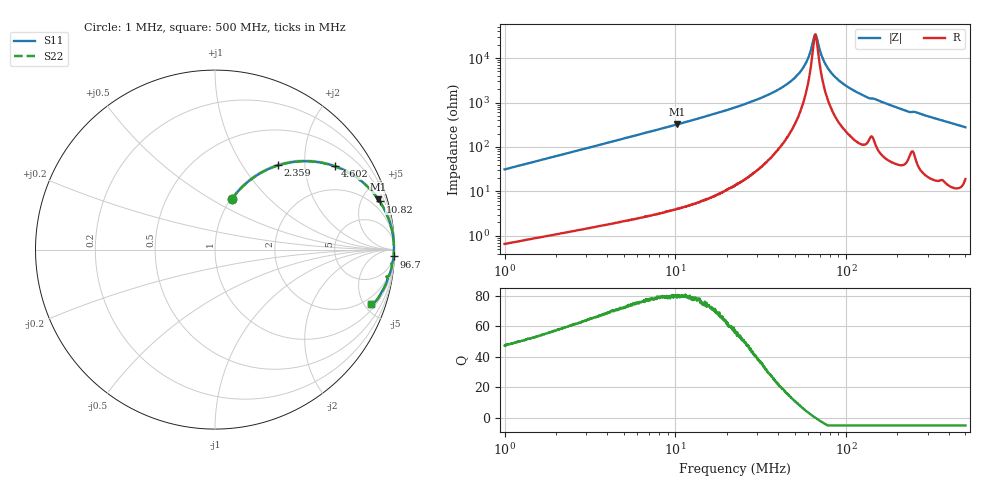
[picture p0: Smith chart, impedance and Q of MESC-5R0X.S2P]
!s-Parameter Generated by FASTRON Sdn. Bhd.
!FASTRON P/N : MESC-5R0X
!Keysight Technologies,E4991B,MY54100416,A.01.15
!Date: Mon Mar 16 10:51:36 2026
!Version  : Rev00 Mon Mar 16 10:51:36 2026
!Data & Calibration Information:
!PortZ  Port1:50+j0  Port2:50+j0
!When reading, reference impedance value at option line is always used.
! Remarks : This data is being provided solely for informational purposes.
!Freq	S11	S21	S12	S22
# Hz S dB R 50
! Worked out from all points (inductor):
!   1601 points, 1 MHz to 500 MHz, reference 50 ohm
!   read as one part in series: L = 4.97 uH near 1.032 MHz
!   highest Q = 80.4 at 10.28 MHz (marker M1), where L = 5.01 uH
!   self-resonance near 66.09 MHz
!   S11 on the Smith chart (normalised r, x): 1 MHz: 1.01, +0.63; 2.359 MHz: 1.02, +1.46; 4.602 MHz: 1.04, +2.85; 10.82 MHz: 1.09, +6.82; 96.7 MHz: 6, -52; 500 MHz: 1.38, -5.55
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1000000  -10.54 71.5  -0.46 -17.3  -0.46 -17.3  -10.54 71.5
2359366  -4.64 53.2  -1.93 -35.9  -1.93 -35.9  -4.64 53.2
2820919  -3.70 48.3  -2.54 -40.8  -2.54 -40.8  -3.70 48.3
4601872  -1.79 34.8  -4.88 -54.4  -4.88 -54.4  -1.79 34.8
7957584  -0.69 21.8  -8.59 -67.4  -8.59 -67.4  -0.69 21.8
1.028286e7  -0.43 17.1  -10.63 -72.2  -10.63 -72.2  -0.43 17.1
1.081541e7  -0.39 16.3  -11.05 -73.0  -11.05 -73.0  -0.39 16.3
2.236068e7  -0.09 7.3  -17.88 -81.7  -17.88 -81.7  -0.09 7.3
3.508814e7  -0.04 3.8  -23.57 -84.3  -23.57 -84.3  -0.04 3.8
4.713694e7  -0.03 1.9  -29.42 -83.9  -29.42 -83.9  -0.03 1.9
5.657749e7  -0.02 0.9  -36.17 -79.4  -36.17 -79.4  -0.02 0.9
6.020511e7  -0.02 0.5  -40.36 -72.8  -40.36 -72.8  -0.02 0.5
6.307767e7  -0.02 0.3  -45.31 -58.4  -45.31 -58.4  -0.02 0.3
6.506845e7  -0.02 0.1  -49.67 -29.2  -49.67 -29.2  -0.02 0.1
6.660267e7  -0.03 -0.0  -50.43 12.6  -50.43 12.6  -0.03 -0.0
7.254416e7  -0.03 -0.5  -40.37 70.6  -40.37 70.6  -0.03 -0.5
7.719553e7  -0.03 -0.9  -36.17 76.8  -36.17 76.8  -0.03 -0.9
8.47377e7  -0.03 -1.4  -32.13 80.6  -32.13 80.6  -0.03 -1.4
9.670074e7  -0.04 -2.2  -28.34 82.2  -28.34 82.2  -0.04 -2.2
1.314291e8  -0.08 -4.2  -22.58 80.7  -22.58 80.7  -0.08 -4.2
1.77937e8  -0.11 -6.3  -19.19 80.6  -19.19 80.6  -0.11 -6.3
5e8  -0.71 -19.3  -9.60 66.8  -9.60 66.8  -0.71 -19.3
